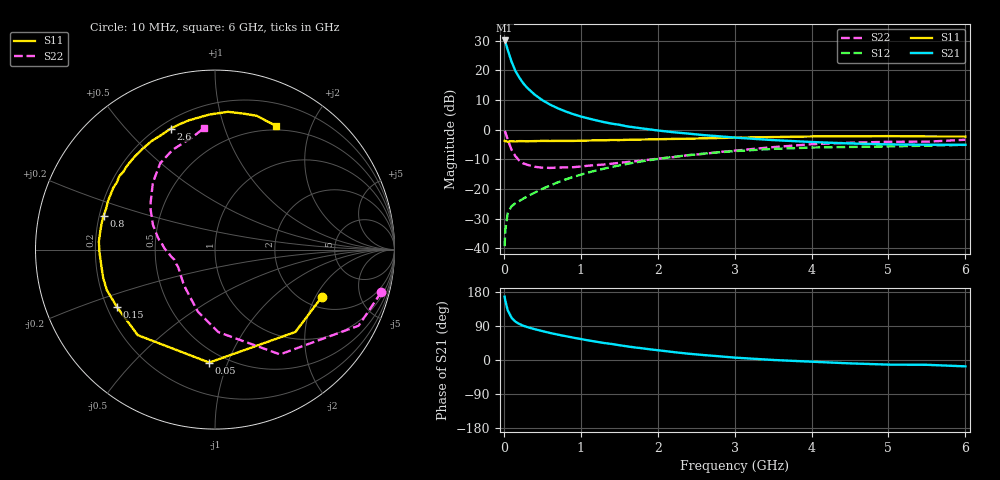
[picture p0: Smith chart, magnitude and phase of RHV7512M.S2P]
! SIEMENS Small Signal Semiconductors
! BFR106
! Si NPN RF Bipolar Junction Transistor in SOT23
! VCE = 0.75 V  IC = 12 mA
! Common Emitter S-Parameters:  August  1996
# GHz  S  MA  R  50
!  f  S11  S21  S12  S22
! GHz  MAG  ANG  MAG  ANG  MAG  ANG  MAG  ANG
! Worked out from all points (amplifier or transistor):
!   36 points, 10 MHz to 6 GHz, reference 50 ohm
!   highest |S21| = 30.1 dB at 10 MHz (marker M1)
!   |S21| within 3 dB of that: start of sweep to 48.41 MHz
!   unconditionally stable (mu >= 1): 412 MHz to end of sweep
!   at 250 MHz: K = 0.79, MSG = 19.5 dB, |S12| = -23.3 dB
!   at 1.4 GHz: K = 1.12, MAG = 5.2 dB, |S12| = -12.6 dB
!   at 6 GHz: K = 1.03, MAG = -1.1 dB, |S12| = -5.1 dB
!   S11 on the Smith chart (normalised r, x): 10 MHz: 2.48, -2.26; 50 MHz: 0.41, -0.86; 150 MHz: 0.24, -0.26; 800 MHz: 0.22, +0.14; 2.6 GHz: 0.24, +0.67; 6 GHz: 0.45, +1.51
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0.01  0.6516 -23.8  32.02 167.0  0.0109 81.5  0.9561 -14.4
0.02  0.6412 -45.7  30.03 156.2  0.0207 69.9  0.9058 -27.9
0.05  0.6302 -92.9  22.31 131.4  0.0392 52.1  0.687 -58.2
0.1  0.6423 -132.1  14.06 111.6  0.0514 41.8  0.4599 -87.7
0.15  0.6328 -149.5  9.871 101.4  0.0577 40.1  0.3591 -105.3
0.2  0.6436 -159.5  7.613 95.3  0.0627 42.2  0.3025 -116.7
0.25  0.6425 -165.9  6.13 90.6  0.0687 43.9  0.2721 -126.9
0.3  0.6397 -171.0  5.15 87.2  0.0745 46.6  0.2576 -133.2
0.4  0.6438 -178.7  3.917 81.4  0.0871 50.4  0.2379 -143.8
0.5  0.6486 176.0  3.158 76.3  0.1008 53.0  0.2293 -151.0
0.6  0.6472 171.0  2.657 71.4  0.1148 54.4  0.2272 -155.5
0.7  0.6484 166.7  2.308 67.0  0.1296 55.6  0.2301 -159.3
0.8  0.6488 163.1  2.041 63.0  0.1447 55.7  0.2324 -163.3
1.1  0.6581 151.9  1.55 51.6  0.1903 55.0  0.2478 -171.0
1.3  0.6627 145.6  1.346 45.0  0.2208 53.1  0.2592 -176.0
1.6  0.6763 136.8  1.141 36.0  0.2651 49.7  0.2853 177.5
2.2  0.7006 120.2  0.909 21.0  0.3483 41.0  0.3452 163.3
2.6  0.7177 110.2  0.811 13.0  0.3957 34.5  0.3927 153.4
3.5  0.7531 92.4  0.669 0.1  0.4756 19.9  0.5094 132.8
4.5  0.774 78.2  0.587 -8.9  0.5132 5.5  0.6043 112.9
5.5  0.7708 67.6  0.559 -12.7  0.5392 -3.3  0.6297 103.1
6  0.7688 63.8  0.557 -16.8  0.5552 -9.7  0.678 95.4
